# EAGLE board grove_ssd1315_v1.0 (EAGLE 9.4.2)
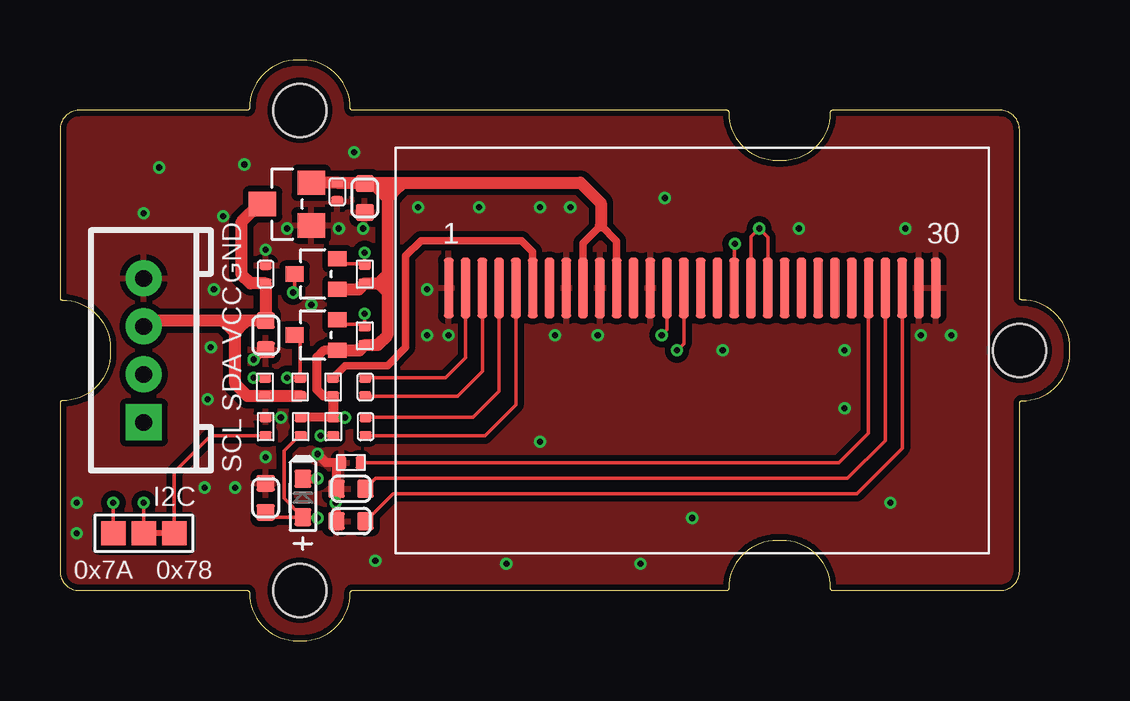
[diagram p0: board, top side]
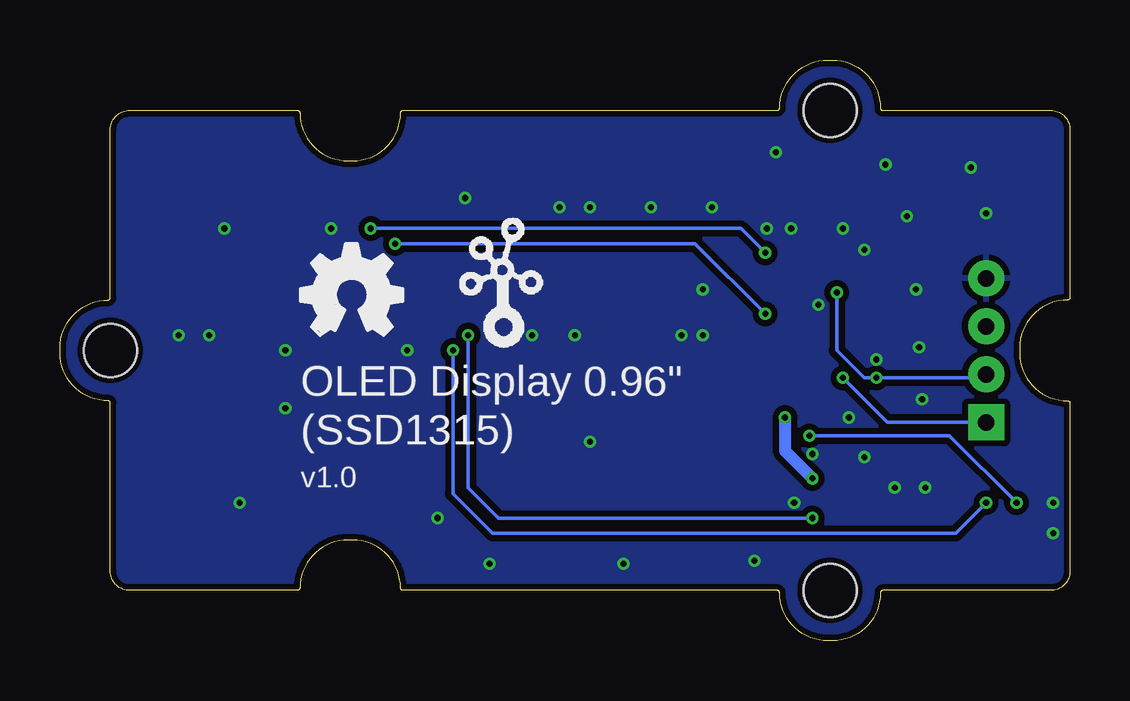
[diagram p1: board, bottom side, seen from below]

Size 42.1 x 24.2 mm. Coordinates in mm from the lower left corner, seen from the top.
Copper layers (1*16): Top 0.035mm / dielectric 1.5mm / Bottom 0.035mm
Design rules "SeeedStudio_2layer_DRU_no_angle_20140221": minimum track width 1mil, minimum drill 10mil, track to track 6mil, track to pad 6mil, pad to pad 6mil, via to via 6mil, smd to smd 0mil, copper to edge 10mil, drill to drill 10mil, minimum pad ring 4mil, minimum via ring 4mil, stop-mask expansion 2mil, vias tented up to drill 25mil, thermal gap 10mil
Net classes: 0 default: width 0.152 mm, drill 0.254 mm, clearance 0.152 mm; 1 power: width 0.152 mm, drill 0.254 mm, clearance 0.152 mm; 2 gnd: width 0.152 mm, drill 0.254 mm, clearance 0.152 mm; 3 usbvcc: width 0.152 mm, drill 0.254 mm, clearance 0.152 mm
bRestrict: area 36.4,-10.9 to 36.8,-10.6; area 27.4,-15 to 27.8,-14.4; area 25,-15 to 26,-14.4; area 18.9,-15 to 21.2,-14.4; area 14.2,-11 to 14.6,-10.5

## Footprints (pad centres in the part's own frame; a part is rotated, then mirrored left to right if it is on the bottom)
C0603 = smd 0.696 x 0.762: 1 0.602,0; 2 -0.602,0
C0402 = smd 0.385 x 0.508: 1 0.383,0; 2 -0.383,0
SOD-523 = smd 0.762 x 0.7: + 0.8,0; - -0.8,0
HW4-2.0 = drill 0.7 pad 1.5 square: 1 -3,0 | drill 0.7 pad 1.5: 2 -1,0; 3 1,0; 4 3,0
3P-SMD-SHORT = smd 1.016 x 1.016: 00 -1.27,0; 11 1.27,0; MM 0,0
SOT-323 = smd 0.762 x 0.635: 1 0.889,-0.635; 2 0.889,0.635; 3 -0.889,0
R0402 = smd 0.385 x 0.508: 1 0.383,0; 2 -0.383,0
SOT-23 = smd 1.016 x 1.143: 1 -0.889,-1.016; 2 0.889,-1.016; 3 0,1.016
OLED30P-0.7-24.74X16.9MM = smd 0.4 x 2.5: 1 -10.15,2.604; 2 -9.45,2.604; 3 -8.75,2.604; 4 -8.05,2.604; 5 -7.35,2.604; 6 -6.65,2.604; 7 -5.95,2.604; 8 -5.25,2.604; 9 -4.55,2.604; 10 -3.85,2.604; 11 -3.15,2.604; 12 -2.45,2.604; 13 -1.75,2.604; 14 -1.05,2.604; 15 -0.35,2.604; 16 0.35,2.604; 17 1.05,2.604; 18 1.75,2.604; 19 2.45,2.604; 20 3.15,2.604; 21 3.85,2.604; 22 4.55,2.604; 23 5.25,2.604; 24 5.95,2.604; 25 6.65,2.604; 26 7.35,2.604; 27 8.05,2.604; 28 8.75,2.604; 29 9.45,2.604; 30 10.15,2.604
2U-DIM-W/DRILL = hole 2.2: -10,-10; -10,10; 20,0

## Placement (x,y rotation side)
C1  10uF/10V  [C0603]  8.58,12.73 90 top
C2  10uF/10V  [C0603]  12.71,18.45 90 top
C3  1uF  [C0402]  12.73,10.58 270 top
C4  1uF  [C0402]  12.74,8.93 270 top
C5  10uF  [C0603]  8.57,5.95 270 top
C6  4.7uF/10V  [C0603]  12.13,6.33 180 top
C7  2.2uF/10V  [C0603]  12.13,4.99 180 top
C8  100nF  [C0402]  8.57,15.27 90 top
C9  100nF  [C0402]  11.56,18.7 270 top
D1  1N4148WT  [SOD-523]  10.12,5.95 270 top
FR1  SEEEDSTUDIO-OPEN-SCH-FRAME  [SEEEDSTUDIO-PCB-FRAME]  not placed on the board
FR2  SEEEDSTUDIO-OPEN-SCH-FRAME  [SEEEDSTUDIO-PCB-FRAME]  not placed on the board
J1  [HW4-2.0]  3.49,12.1 90 top
JP1  [3P-SMD-SHORT]  3.49,4.48 0 top
LOGO1  LOGO-OSHW-FILLX0150-NT  [OSHW_FILLX150_NOTEXT]  32.07,12.73 0 bottom
Q3  CJ2102  [SOT-323]  10.67,15.28 0 top
Q4  CJ2102  [SOT-323]  10.67,12.74 0 top
R1  4.7k  [R0402]  12.71,15.27 270 top
R2  4.7k  [R0402]  12.71,12.71 90 top
R3  4.7k  [R0402]  8.54,10.58 90 top
R4  4.7k  [R0402]  10.01,10.58 90 top
R5  4.7k  [R0402]  10.04,8.93 270 top
R6  0R  [R0402]  11.38,10.58 270 top
R7  4.7k  [R0402]  8.57,8.93 90 top
R8  620k  [R0402]  12.13,7.43 0 top
R9  4.7k  [R0402]  11.39,8.93 90 top
U1  XC6206P332MR  [SOT-23]  9.46,18.2 90 top
U4  [OLED30P-0.7-24.74X16.9MM]  26.35,12.1 0 top
U5  [2U-DIM-W/DRILL]  20,12.1 0 top
U$1  LOGO-GROVETWIGLOGO_SMALL  [GROVE-SILK-SMALL]  25.85,12.1 0 bottom

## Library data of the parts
C1-C9 R1-R9 = Discrete-small
D1 JP1 Q3 Q4 = Discrete-new
FR1 FR2 U4 = moudle-new
J1 = Connector-new
LOGO1 U$1 = logo; PARTNO: DNP
U1 = IC-new
U5 = moudle

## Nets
3V3: C2.1 C9.2 D1.- Q3.1 Q4.1 R1.1 R2.2 R5.2 R6.1 R9.1 U1.2 U4.9 U4.11
GND: C1.2 C2.2 C5.2 C6.1 C7.1 C8.1 C9.1 J1.4 R7.1 R8.2 U1.1 U4.1 U4.8 U4.10 U4.13 U4.29 U4.30
HSCL: J1.1 Q4.3 R4.1
HSDA: J1.2 Q3.3 R3.1
IIC_ADDR: JP1.MM U4.15
N$1: C3.2 U4.2
N$2: C4.2 U4.4
N$3: C3.1 U4.3
N$4: C4.1 U4.5
N$5: R8.1 U4.26
N$6: C6.2 U4.27
N$7: C7.2 U4.28
N$8: R6.2 U4.6
N$10: JP1.11 R7.2
N$11: JP1.00 R9.2
RES: C5.1 D1.+ R5.1 U4.14
SCL: Q4.2 R2.1 U4.18
SDA: Q3.2 R1.2 U4.19 U4.20
VCC_IN: C1.1 C8.2 J1.3 R3.2 R4.2 U1.3

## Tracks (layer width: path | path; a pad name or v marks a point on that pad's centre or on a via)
3V3  (via drill 0.25 pad 0.51)
  Top 0.152: 12.67,19.09 13.53,19.09 13.65,18.96
  Top 0.305: U4.9 21.8,16.57 22.54,17.31 23.2,16.65 U4.11
  Top 0.381: v11.88,9.31 11.75,9.31 R9.1 R5.2 | D1.- 10.72,6.75 v10.73,6.77 | R6.1 10.98,10.19 10.71,10.47 10.71,11.82 10.99,12.1 Q4.1
  Top 0.406: R6.1 11.38,9.32 R9.1
  Top 0.508: Q3.1 12.46,14.64 R1.1 12.99,14.89 13.27,14.89 | Q4.1 12.48,12.1 R2.2 13.25,12.33 13.65,12.73 13.65,14.51 | U1.2 C9.2 12.67,19.09 | 12.67,19.09 C2.1 | 12.67,19.09 21.69,19.09 22.54,18.23 22.54,17.31 | 13.65,18.96 13.65,18.45 | 13.65,18.45 13.65,15.27 | 13.65,15.27 13.65,15.02 | 13.65,15.02 13.65,14.51 | 13.27,14.89 13.53,14.89 13.65,15.02 | 13.65,18.45 13.02,19.09 | 13.65,18.45 14.16,18.96 | 13.27,14.89 13.65,15.27 | 13.27,14.89 13.28,14.89 13.65,14.51
  Bottom 0.508: v11.88,9.31 11.88,7.91 v10.73,6.77
GND  (via drill 0.25 pad 0.51)
  Top 0.381: R8.2 11.09,7.43 v10.73,7.78 | C1.2 8.48,12.13 v8.07,11.72 | C7.1 11.53,7.37 11.5,7.4
  Top 0.508: C6.1 11.53,6.43
  other vias: 3.49,17.81 0.7,4.48 4.13,19.72 7.69,19.85 6.8,17.69 6.42,14.64 6.29,12.23 6.16,10.07 6.03,6.38 15.31,14.64 25.21,18.45 13.15,3.34 18.61,3.21 24.2,3.21 26.35,5.11 9.21,9.31 8.57,7.65 11.5,5.75 8.57,16.29 11.62,17.18 12.64,17.18 0.7,5.75 12.26,20.36 9.46,17.18 7.3,6.38 16.19,12.73 15.31,12.73 21.27,18.07 20,18.07 20.64,12.73 22.42,12.73 35.88,12.73 37.15,12.73 27.62,12.1 32.7,12.1 20,8.29 34.61,5.75 32.7,9.69 30.8,17.18 35.24,17.18 14.92,18.07 17.46,18.07 10.48,14
  pour Bottom (isolate 0.254): -0.32,24.16 42.23,24.16 42.23,1.94 42.23,0.04 -0.32,0.04
  pour Top (isolate 0.254): -0.32,24.16 42.23,24.16 42.23,1.94 42.23,0.04 -0.32,0.04
HSCL  (via drill 0.25 pad 0.51)
  Top 0.152: v9.46,10.96 v9.47,10.96 R4.1 10.01,12.51 Q4.3
  Bottom 0.152: J1.1 7.61,9.1 v9.46,10.96
HSDA  (via drill 0.25 pad 0.51)
  Top 0.152: R3.1 v8.07,10.96 | Q3.3 9.78,14.58 v9.72,14.51
  Bottom 0.152: v9.72,14.51 9.72,12.1 8.57,10.96 v8.07,10.96 3.19,10.96 J1.2
IIC_ADDR  (via drill 0.25 pad 0.51)
  Top 0.152: JP1.MM v3.49,5.75 | U4.15 26,12.38 v25.72,12.1
  Bottom 0.152: v3.49,5.75 4.76,4.48 24.07,4.48 25.72,6.13 v25.72,12.1
N$1
  Top 0.152: C3.2 16.07,10.96 16.9,11.79 U4.2
N$2
  Top 0.152: C4.2 17.21,9.31 18.3,10.4 U4.4
N$3
  Top 0.152: C3.1 16.57,10.19 17.6,11.22 U4.3
N$4
  Top 0.152: C4.1 17.72,8.54 18.61,9.43 18.73,9.56 19,9.83 U4.5
N$5
  Top 0.152: R8.1 32.48,7.43 32.7,7.65 33.34,8.29 33.7,8.65 U4.26
N$6
  Top 0.152: U4.27 34.4,8.34 32.83,6.77 13.16,6.77 C6.2
N$7
  Top 0.152: U4.28 35.1,8.02 33.21,6.13 13.88,6.13 C7.2
N$8
  Top 0.305: R6.2 11.89,11.46 13.65,11.46 14.42,12.23 14.42,16.04 15.05,16.67 19.24,16.67 19.7,16.21 U4.6
N$10
  Top 0.152: R7.2 6.29,8.54 4.76,7.02 JP1.11
N$11  (via drill 0.25 pad 0.51)
  Top 0.152: R9.2 v10.86,8.54 | JP1.00 v2.22,5.75
  Bottom 0.152: v10.86,8.54 5.02,8.54 v2.22,5.75
RES  (via drill 0.25 pad 0.51)
  Top 0.152: D1.+ 10.7,5.15 v10.73,5.11 | D1.+ 8.77,5.15 C5.1 | U4.14 25.3,12.96 v25.08,12.73 | R5.1 9.97,8.54 9.34,7.91 9.34,5.94 D1.+
  Bottom 0.152: v25.08,12.73 25.08,6.38 23.81,5.11 v10.73,5.11
SCL  (via drill 0.25 pad 0.51)
  Top 0.152: U4.18 28.1,16.52 v28.13,16.55 | v12.7,13.62 12.7,13.18 | 12.7,13.18 R2.1 12.66,13.09 12.64,13.12 12.7,13.18 | 12.7,13.18 11.75,13.18 Q4.2
  Bottom 0.152: v28.13,16.55 15.62,16.55 v12.7,13.62
SDA  (via drill 0.25 pad 0.51)
  Top 0.152: v12.7,16.16 12.71,16.1 R1.2 12.64,15.72 11.75,15.72 Q3.2 | U4.19 28.8,16.84 v29.15,17.18 29.5,16.82 U4.20
  Bottom 0.152: v29.15,17.18 13.72,17.18 v12.7,16.16
VCC_IN
  Top 0.152: 7.3,12.86 7.27,12.86 7.16,12.97
  Top 0.508: U1.3 8.32,18.2 7.56,17.43 7.56,15.27 7.94,14.89 C8.2 C1.1 6.8,13.34 | R4.2 R3.2 7.81,10.19 7.3,10.7 7.3,12.83 | 7.3,12.83 7.3,12.86 | 7.3,12.86 7.3,13.24 | 6.8,13.34 3.73,13.34 J1.3 | 7.3,12.83 7.16,12.97 6.8,13.34 | 7.3,12.73 7.3,12.83 | 7.3,12.86 7.69,13.24

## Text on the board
tPlace: GND | VCC | SDA | SCL | I2C | 0x7A | 0x78
bPlace: OLED Display 0.96" | (SSD1315) | v1.0

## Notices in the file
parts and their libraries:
moudle-new: This work is licensed under the Creative Commons Attribution 4.0 International License.
To view a copy of this license,visit:
http://creativecommons.org/licenses/by-sa/4.0
